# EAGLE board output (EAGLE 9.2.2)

Size 160 x 100 mm. Coordinates in mm from the lower left corner, seen from the top.
Outline: 0,0 160,0 160,100 0,100 0,0
Copper layers (1*16): Top 0.035mm / dielectric 1.5mm / Bottom 0.035mm
Design rules "default *": minimum track width 6mil, minimum drill 0.35mm, track to track 16mil, track to pad 16mil, pad to pad 16mil, via to via 16mil, smd to smd 16mil, copper to edge 40mil, drill to drill 6mil, minimum pad ring 10mil, minimum via ring 8mil, stop-mask expansion 4mil, vias tented up to drill 0mil, thermal gap 10mil

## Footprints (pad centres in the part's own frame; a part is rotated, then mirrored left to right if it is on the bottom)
R1206FAB = smd 1.27 x 1.905: 1 -1.651,0; 2 1.651,0
C1206FAB = smd 1.27 x 1.905: 1 -1.651,0; 2 1.651,0
SOIC14 = smd 0.61 x 2.21: 1 -3.81,-2.603; 2 -2.54,-2.603; 3 -1.27,-2.603; 4 0,-2.603; 5 1.27,-2.603; 6 2.54,-2.603; 7 3.81,-2.603; 8 3.81,2.603; 9 2.54,2.603; 10 1.27,2.603; 11 0,2.603; 12 -1.27,2.603; 13 -2.54,2.603; 14 -3.81,2.603
2X03SMD = smd 2.54 x 1.27: 1 -2.54,2.54; 2 2.92,2.54; 3 -2.54,0; 4 2.92,0; 5 -2.54,-2.54; 6 2.92,-2.54
1X06SMD = smd 2.54 x 1.27: 1 0,6.35; 2 0,3.81; 3 0,1.27; 4 0,-1.27; 5 0,-3.81; 6 0,-6.35
EFOBM = smd 0.8 x 3.9: 1 -1.35,0; 2 0,0; 3 1.35,0
2X02SMD = smd 2.54 x 1.27: 1 -2.54,1.27; 2 2.92,1.27; 3 -2.54,-1.27; 4 2.92,-1.27
P-LCC-4-3 = smd 1.1 x 1.5: A -0.8,1.5; B 0.8,1.5; G 0.8,-1.5; R -0.8,-1.5

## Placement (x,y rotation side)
B  499  [R1206FAB]  64.77,73.66 0 top
C1  1UF  [C1206FAB]  58.42,71.12 0 top
G  499  [R1206FAB]  67.31,49.53 0 top
IC1  ATTINY44-SSU  [SOIC14]  58.42,63.5 270 top
R  1k  [R1206FAB]  64.77,69.85 0 top
R2  10K  [R1206FAB]  44.45,66.04 90 top
U$1  AVRISPSMD  [2X03SMD]  58.42,52.07 270 top
U$2  FTDI-SMD-HEADER  [1X06SMD]  80.01,66.04 0 top
U$3  RESONATOR  [EFOBM]  49.53,66.04 90 top
U$4  PINHD-2X2-SMD  [2X02SMD]  71.12,57.15 0 top
U$5  [P-LCC-4-3]  71.12,68.58 0 top

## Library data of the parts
B C1 G IC1 R R2 U$1-U$5 = fab

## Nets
A0: IC1.5
B: B.1
G: G.1
GND: C1.1 IC1.14 U$1.6 U$2.1 U$3.2 U$4.3
MISO: IC1.8 U$1.1 U$4.2
MOSI: IC1.7 U$1.4
N$1: R.2 U$5.R
N$2: B.2 U$5.B
N$3: G.2 U$5.G
R: R.1
R1: IC1.10
R2: IC1.11
R3: IC1.6
RESET: IC1.4 R2.1 U$1.5
RXD: IC1.12 U$2.5
SCK: IC1.9 U$1.3 U$4.4
TXD: IC1.13 U$2.4
VCC: C1.2 IC1.1 R2.2 U$1.2 U$2.3 U$4.1 U$5.A
XTAL1: IC1.2 U$3.1
XTAL2: IC1.3 U$3.3

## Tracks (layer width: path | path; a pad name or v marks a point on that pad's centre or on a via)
GND  (5 unrouted)
MISO  (2 unrouted)
MOSI  (1 unrouted)
N$1  (1 unrouted)
N$2  (1 unrouted)
N$3  (1 unrouted)
RESET  (2 unrouted)
RXD  (1 unrouted)
SCK  (2 unrouted)
TXD  (1 unrouted)
VCC  (6 unrouted)
XTAL1  (1 unrouted)
XTAL2  (1 unrouted)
